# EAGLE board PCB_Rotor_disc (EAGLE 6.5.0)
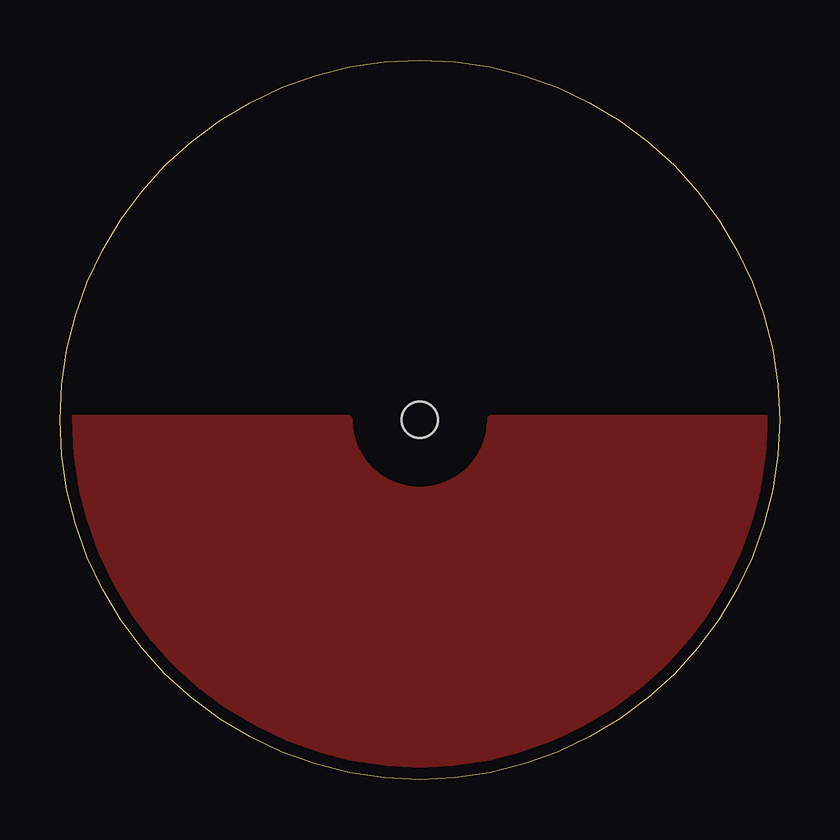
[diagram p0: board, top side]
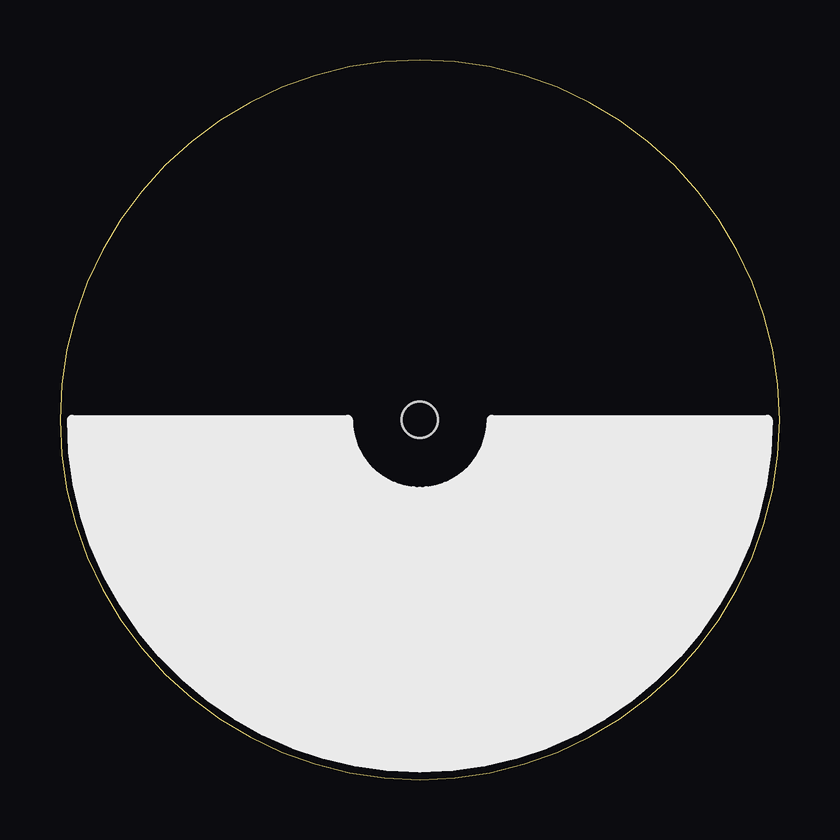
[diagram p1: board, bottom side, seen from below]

Size 30 x 30 mm. Coordinates in mm from the lower left corner, seen from the top.
Outline: 0,15 arc-180 30,15 arc-180 0,15
Copper layers (1*16): Top 0.035mm / dielectric 1.5mm / Bottom 0.035mm
Design rules "default *": minimum track width 10mil, minimum drill 24mil, track to track 8mil, track to pad 8mil, pad to pad 8mil, via to via 8mil, smd to smd 8mil, copper to edge 0.5mm, drill to drill 8mil, minimum pad ring 10mil, minimum via ring 8mil, stop-mask expansion 4mil, vias tented up to drill 0mil, thermal gap 10mil
Holes 1.5 mm at 15,15

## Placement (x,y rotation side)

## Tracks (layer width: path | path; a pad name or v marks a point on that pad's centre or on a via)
S$1
  pour Top: 0,15 arc90 15,0 arc90 30,15 18,15 arc-90 15,12 arc-90 12,15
